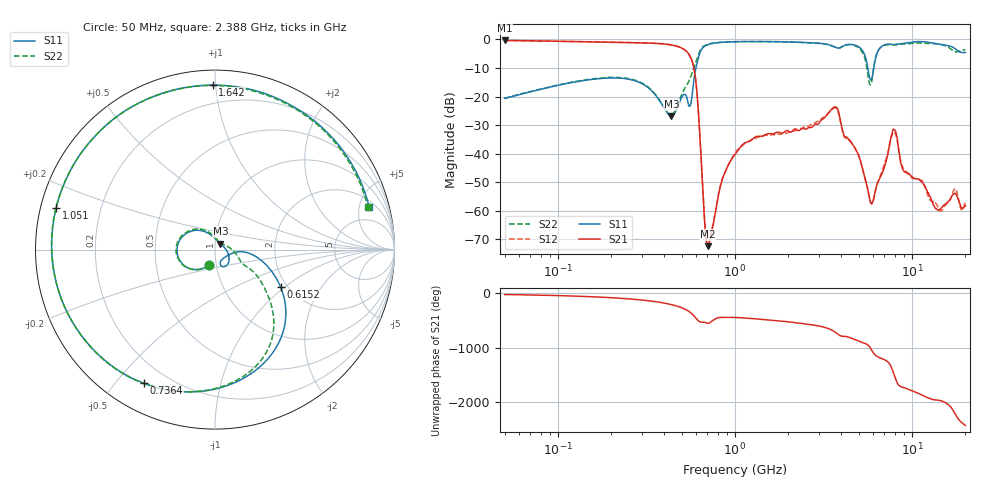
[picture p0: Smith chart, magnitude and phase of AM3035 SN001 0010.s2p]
# Hz S DB R 50
!freq MagS11 AngS11 MagS21 AngS21 MagS12 AngS12 MagS22 AngS22
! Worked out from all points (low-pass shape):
!   1601 points, 50 MHz to 20.05 GHz, reference 50 ohm
!   highest |S21| = -0.36 dB at 50 MHz (marker M1); lowest = -72.4 dB at 704.1 MHz (marker M2)
!   |S21| within 3 dB of the highest: start of sweep to 512 MHz
!   lowest |S11| = -26.9 dB at 437.5 MHz (marker M3), VSWR 1.09, Z = 53 + j3.58 ohm
!   |S11| at or under -10 dB: start of sweep to 602.2 MHz; 5.635 GHz to 6.088 GHz (452.5 MHz wide, 7.72 % of centre)
!   |S22| runs from -26.4 to -0.7 dB; largest |S21 - S12| = 0.0048
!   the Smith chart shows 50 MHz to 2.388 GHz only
!   S11 on the Smith chart (normalised r, x): 50 MHz: 0.92, -0.16; 615.2 MHz: 1.84, -0.94; 736.4 MHz: 0.11, -0.59; 1.051 GHz: 0.05, +0.13; 1.642 GHz: 0.09, +0.98; 2.388 GHz: 2.70, +6.23
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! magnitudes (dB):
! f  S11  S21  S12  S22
! 50 MHz  -20.6  -0.4  -0.4  -20.6
! 135.9 MHz  -14.5  -0.8  -0.8  -14.3
! 369.6 MHz  -20.8  -1.4  -1.4  -20.7
! 437.5 MHz  -26.9  -1.9  -1.9  -26.4
! 560.2 MHz  -23.0  -6.1  -6.1  -13.4
! 615.2 MHz  -7.5  -21.2  -21.1  -6.2
! 675.6 MHz  -2.4  -64.6  -64.2  -2.1
! 704.1 MHz  -1.8  -72.4  -72.0  -1.7
! 736.4 MHz  -1.5  -67.9  -67.6  -1.4
! 1.005 GHz  -0.8  -40.1  -39.7  -0.8
! 1.051 GHz  -0.8  -38.4  -38.3  -0.8
! 1.642 GHz  -0.8  -33.0  -33.4  -0.8
! 2.388 GHz  -1.0  -31.2  -31.1  -1.1
! 2.722 GHz  -1.2  -30.8  -29.9  -1.2
! 3.743 GHz  -2.9  -23.7  -24.2  -2.9
! 5.013 GHz  -2.6  -40.9  -40.7  -3.0
! 5.912 GHz  -14.0  -57.4  -57.6  -15.1
! 7.402 GHz  -1.6  -38.2  -38.4  -1.8
! 8.008 GHz  -1.8  -31.7  -32.8  -1.9
! 8.927 GHz  -1.4  -45.8  -45.1  -1.6
! 13.84 GHz  -1.5  -59.5  -57.9  -1.5
! 20.05 GHz  -4.5  -58.1  -57.2  -3.6
